PROGRAM Cutter
VAR
	
	//运动控制指令
	FB_MasterPower,FB_SlavePower      : MC_Power;          //使能
	FB_MasterMoveVelo                 : MC_MoveVelocity;   //匀速运动
    FB_SlaveMoveMo                    : MC_MoveModulo;     //模值绝对定位
	FB_SetMasterPos                   : MC_SetPosition;    //设定主轴位置
	FB_MasterHalt                     : MC_Halt;           //主轴停止
	FB_MasterReset,FB_SlaveReset      : MC_Reset;          //主从轴复位
	b_MasterReset,b_SlaveReset        : BOOL;              
	b_SetMasterPos                    : BOOL;
	b_SlavePower,b_MasterPower        : BOOL;
	b_CutterReset                     : BOOL;

	
	//电子凸轮
	FB_CreatCamTable                  : MC_CamTableSelect; //创建凸轮表功能块
	CutterTable                       : ARRAY[1..3] OF MC_MotionFunctionPoint; //关键点定义
	CutterCam_Ref                     : MC_CAM_REF;        //凸轮变量
	FB_CamIn                          : MC_CamIn;          //耦合功能块
	FB_CamOut                         : MC_CamOut;         //解耦功能块
	b_CreatTable                      : BOOL;
	b_StartCut                  AT %I*: BOOL;
	b_CamOut                          : BOOL;
	b_HomeSlave                       : BOOL;
	
    //其它
	SlaveHomingStep                   : INT;               //旋刀回零步
	CutterStep                        : INT;               //旋切步
	IsSlaveReady                      : BOOL;              //从轴是否准备完成
 	IsMasterReady                     : BOOL;              //主轴是否准备完成
	IsAxisError                       : BOOL;              //轴是否有报错
	MasterPos                         : ARRAY [1..PointNumber] OF LREAL := [0.0,105 , 180];
	SlavePos                          : ARRAY[1..PointNumber] OF LREAL := [0.0,90, 180];
	
	
	CutterDistance1,CutterDistance2	  :	LREAL;    //队列用距离计算 1用于旋切触发 2用于皮带启停
	bpopCutter1,bpopCutter2			  : BOOL;     //队列用标志位
	Delay                             : Ton;
	BeltStep                          : INT;     //皮带启停Case步

	//出料
	FB_MoveReMaster                   : MC_MoveRelative; 
	MatrialOutStep                    : INT;    
	MaterialOut                       : BOOL;   
END_VAR
VAR CONSTANT
	PointNumber                       : LINT := 3;  //关键点数量         
END_VAR

//调用耦合、解耦功能块
CamIn_and_Out();
//调用凸轮表
CamTable();
//调用运动控制功能块和回零功能
MotionCommand();
//调用皮带启停逻辑
BeltCommand();

//读取主、从轴状态
Cutter_Master.ReadStatus();
Cutter_Slave.ReadStatus();


//旋切逻辑
CASE CutterStep OF 
0://触发位复位
  b_CreatTable     :=FALSE;   
  b_StartCut       :=FALSE;
  b_CamOut         :=FALSE;
  CutterStep       :=1;
  //MaterialNum      :=0;
  
1: //创建凸轮表
   b_CreatTable :=TRUE;
   IF FB_CreatCamTable.Done THEN
	   b_CreatTable :=FALSE;
	   CutterStep:=5;
   END_IF
   IF  FB_CreatCamTable.error THEN
	   b_CreatTable :=FALSE;
	   CutterStep:=99;
   END_IF
   
5: 
//gCurrentCutterEnc:=gCurrentCutterEncNull;
//CutterDistance:=gCurrentCutterEncNull;
//比较队列中的数据是否为空，不为空则允许取
  IF (MEMCMP(pBuf1:=ADR(garrayCutterenc1[1]) , pBuf2:=ADR(gCurrentCutterEncNull1) , n:=SIZEOF(gCurrentCutterEncNull1) )<>0) THEN
      bpopcutter1:=TRUE; //允许取标志位
      CutterStep:=6;
  END_IF

6:
//若未在存数据且允许取则取
  IF NOT gbPushPopCutterBusy1 AND bpopcutter1 THEN
		 gfbPushPopCutter1.PopStack();
		 bpopCutter1	:=	FALSE;//允许取标志位复位
  END_IF
  //将队列中的数据赋值到变量中
  gfbPushPopCutter1(ArrayCutterenc:=gArrayCutterenc1 , PushCutterenc:= , PopCutterenc=> gCurrentCutterEnc1, busy=>gbPushPopCutterBusy1 );
 //若变量中已有数据则继续旋切
  IF gCurrentCutterEnc1<>0 THEN
	 CutterStep:=10;
  END_IF
	
10: //判断物料移动的距离
	CutterDistance1:=Cutter_Master.NcToPlc.ActPos-gCurrentCutterEnc1;
	//进入旋切范围则耦合开始旋切
    IF CutterDistance1<=420.5 AND CutterDistance1>=419.5   THEN
	   b_startCut:=TRUE; 
	END_IF
	//若距离大于540且旋刀未移动则代表旋切完成，物料数-1
	IF CutterDistance1>540 AND Cutter_Slave.Status.NotMoving THEN
	   MaterialNum:=MaterialNum-1;
	   CutterStep:=5;
	END_IF
	//耦合则触发位复位
	IF FB_CamIn.InSync THEN   
	   b_StartCut:=FALSE;
	END_IF
	//旋切报错则进入99步
	IF  Cutter_Master.Status.Error OR Cutter_slave.Status.Error  THEN
		b_StartCut:=FALSE;
		CutterStep:=99;
	END_IF
   
99://报错判断步
   //若耦合则解耦
    b_Camout:=Cutter_Slave.Status.Coupled;
	IF NOT Cutter_Slave.Status.Coupled THEN
		   CutterStep:=0;
	END_IF
END_CASE

ACTION BeltCommand:
(*对旋切皮带上是否有物料做判断
  若皮带上有物料则皮带开始运行*)
//判断物料个数，新物料放置则皮带再次启动
IF   MaterialNum>0 AND CutterNum<>MaterialNum THEN
	 FB_MasterMoveVelo.Execute:=TRUE;
END_IF
//若没有物料则停止运行
IF MaterialNum=0 THEN 
   FB_MasterHalt.Execute:=TRUE;
   FB_MasterMoveVelo.Execute:=FALSE;      
END_IF

CASE BeltStep OF
0: 
   FB_MasterHalt.Execute:=FALSE;
   FB_MasterMoveVelo.Execute:=FALSE; 
   //比较队列中是否有数据，有数据则允许取
   IF (MEMCMP(pBuf1:=ADR(garrayCutterenc2[1]) , pBuf2:=ADR(gCurrentCutterEncNull2) , n:=SIZEOF(gCurrentCutterEncNull2) )<>0) THEN
	   bpopcutter2:=TRUE;//取标志位置位
	   BeltStep:=10;
   END_IF

10:
  //若没有在存且取标志位置位则取
   IF NOT gbPushPopCutterBusy2 AND bpopcutter2 THEN
		  gfbPushPopCutter2.PopStack();
		  bpopCutter2	:=	FALSE;
   END_IF
   //将队列中的数据赋值到变量中
   gfbPushPopCutter2(ArrayCutterenc:=gArrayCutterenc2 , PushCutterenc:= , PopCutterenc=> gCurrentCutterEnc2, busy=>gbPushPopCutterBusy2 );
   //若变量中已有数据则继续旋切
   IF gCurrentCutterEnc2<>0 THEN
	  BeltStep:=20;
   END_IF
   
20:
    //计算物料移动的距离 
	CutterDistance2:=Cutter_Master.NcToPlc.ActPos-gCurrentCutterEnc2;
	//到达指定距离后皮带停止
    IF CutterDistance2<=210.5 AND CutterDistance2>=209.5   THEN
	   FB_MasterHalt.Execute:=TRUE;
       FB_MasterMoveVelo.Execute:=FALSE; 
	   AllowToPlace:=TRUE; //允许放置标志位置位
       BeltStep:=0; 	
	END_IF
END_CASE
END_ACTION

ACTION CamIn_and_Out:
//耦合功能块，模式为相对位置
FB_CamIn(
	Master:=Cutter_Master , 
	Slave:=Cutter_Slave, 
	Execute:= b_StartCut, 
	StartMode:=MC_STARTMODE_Relative , 
	SlaveScaling:=-1 , 
	CamTableID:=1 , 
);

//解耦
FB_CamOut(
	Slave:=Cutter_Slave , 
	Execute:=b_CamOut , 
 );
END_ACTION

ACTION CamTable:
//定义凸轮表Action

//创建凸轮表
FB_CreatCamTable(
	Master:=Cutter_Master , 
	Slave:=Cutter_Slave , 
	CamTable:=CutterCam_Ref , 
	Execute:=b_CreatTable , 
	Periodic:=FALSE , 
	CamTableID:=1 , 
 );

//定义凸轮标关键点
CutterCam_Ref.pArray:=ADR(CutterTable);
CutterCam_Ref.ArraySize:=SIZEOF(CutterTable);
CutterCam_Ref.NoOfColumns:=1;
CutterCam_Ref.NoOfRows:=3;
CutterCam_Ref.TableType:=22;

//1号关键点 
CutterTable[1].FunctionType:=3;
CutterTable[1].MasterPos:=MasterPos[1];
CutterTable[1].SlavePos:=SlavePos[1];
CutterTable[1].PointIndex:=1;
CutterTable[1].PointType:=16#0001;

//2号关键点
CutterTable[2].FunctionType:=3;
CutterTable[2].MasterPos:=MasterPos[2];
CutterTable[2].SlavePos:=SlavePos[2];
CutterTable[2].PointIndex:=2;
CutterTable[2].PointType:=16#0002;

//3号关键点
CutterTable[3].FunctionType:=3;
CutterTable[3].MasterPos:=MasterPos[3];
CutterTable[3].SlavePos:=SlavePos[3];
CutterTable[3].PointIndex:=3;
CutterTable[3].PointType:=16#0001;
END_ACTION

ACTION MotionCommand:
//旋刀回零步
CASE SlaveHomingStep OF
0: //触发位复位
   b_HomeSlave:=FALSE;
   b_MasterPower:=FALSE;
   b_SlavePower:=FALSE;
   FB_SlaveMoveMO.Execute:=FALSE;
   SlaveHomingStep:=10;
   
//主轴使能从轴使能
10:
   b_MasterPower:=TRUE;
   b_SlavePower:=TRUE;
   b_HomeSlave:=FALSE;
   IF FB_MasterPower.status AND FB_SlavePower.status THEN
      SlaveHomingStep:=20;
   END_IF
    IF Cutter_Master.Status.Error OR  Cutter_Slave.Status.Error THEN
       SlaveHomingStep:=0;
   END_IF

//从轴回零
20:
   IF b_HomeSlave = TRUE THEN
      FB_SlaveMoveMo.Execute:=TRUE;
	  IF FB_SlaveMoveMO.Done THEN
		 FB_SlaveMoveMo.Execute:=FALSE;
         SlaveHomingStep:=10; 
	  END_IF 
   END_IF 
END_CASE

//出料
CASE MatrialOutStep  OF
0: IF MaterialOut THEN
	  FB_MoveReMaster.Execute:=TRUE;
	  MatrialOutStep:=10;
   END_IF

10:
   IF  FB_MoveReMaster.Done THEN
	   FB_MoveReMaster.Execute:=FALSE;
	   MaterialNum:=0;
	   CutterNum:=0;
	   MatrialOutStep:=0;
   END_IF
END_CASE

//判断主轴状态,若正常则标志位置位
IF FB_MasterPower.status AND NOT Cutter_Master.Status.Error THEN
   IsMasterReady:=TRUE;
   ELSE
   Ismasterready:=FALSE;
END_IF

//判断从轴状态,若正常则标志位置位
IF FB_SlavePower.status AND NOT Cutter_Slave.Status.Error THEN
   IsSlaveReady:=TRUE;
   ELSE
   IsSlaveready:=FALSE;
END_IF

//若报错则标志位置位
IF Cutter_Master.Status.Error OR  Cutter_Slave.Status.Error THEN
   IsAxisError:=TRUE;
END_IF

IF b_CutterReset=TRUE THEN
   b_MasterReset:=TRUE;
   b_SlaveReset:=TRUE;
   IF FB_MasterReset.Done AND FB_SlaveReset.Done THEN
	  FB_SlaveMoveMo.Execute:=FALSE;
	  b_CutterReset:=FALSE;
	  b_MasterReset:=FALSE;
      b_SlaveReset:=FALSE;
	  IsAxisError:=FALSE;
	  MaterialNum:=0;
	  SlaveHomingStep:=0;
   END_IF
END_IF



//读取主从轴状态
Cutter_Master.ReadStatus();
Cutter_Slave.ReadStatus();


//功能块定义部分
FB_MasterPower(
	Axis:=Cutter_Master , 
	Enable:=b_MasterPower , 
	Enable_Positive:=1 , 
	Enable_Negative:=1 , 
 );
 
FB_SlavePower(
	Axis:=Cutter_Slave , 
	Enable:=b_SlavePower , 
	Enable_Positive:=1 , 
	Enable_Negative:=1 , );

//模值绝对定位 
FB_SlaveMoveMo(
	Axis:=Cutter_Slave , 
	Execute:= , 
	Position:=0 , 
	Velocity:=200 , 
);

FB_SetMasterPos(
	Axis:=Cutter_Master , 
	Execute:=b_SetMasterPos , 
	Position:=0 ,  
 );

FB_MasterReset(
	Axis:=Cutter_Master , 
	Execute:=b_MasterReset , 
 );
 
 FB_SlaveReset(
	Axis:=Cutter_Slave , 
	Execute:=b_SlaveReset , 
 );
 
FB_MasterMoveVelo(
	Axis:=Cutter_Master , 
	Execute:= , 
	Velocity:=140 , 
	Direction:= , 
 );
 
 FB_MasterHalt(
	Axis:=Cutter_Master , 
	Execute:= , 
);
 
 FB_MoveReMaster(
	Axis:=Cutter_Master , 
	Execute:= , 
	Distance:=480 , 
	Velocity:=140 , 
 );
END_ACTION

END_PROGRAM
